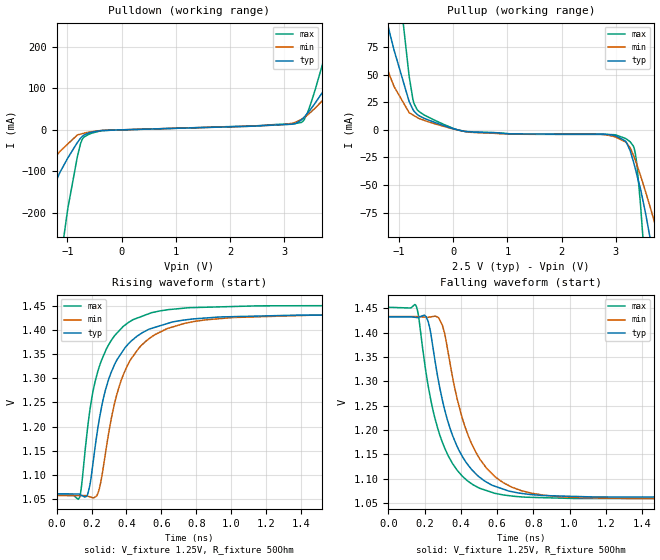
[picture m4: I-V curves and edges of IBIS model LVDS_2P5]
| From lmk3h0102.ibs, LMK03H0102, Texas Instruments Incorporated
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[Model]   LVDS_2P5
Model_type   Output
Polarity   Non-Inverting
Vmeas = 1.25
Vref = 1.25
Cref = 2pF
Rref = 50
|   typ   min   max
C_comp   2.5pF   2pF   3pF
[Voltage Range]   2.5   2.375   2.625
[Temperature Range]   45   125   -40
[Pullup Reference]   2.5   2.375   2.625
[Pulldown Reference]   -0   -0   -0
[Power Clamp Reference]   2.5   2.375   2.625
[GND Clamp Reference]   0   0   0
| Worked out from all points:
|   slope of the pulldown table from 0 to 0.375 V, typ, clamps not added: 278 ohm
|   slope of the pullup table from 0 to 0.375 V, typ, clamps not added: 121 ohm
|   falling waveform, V_fixture 1.25V, R_fixture 50Ohm: 20-80 % time 175ps typ, 189ps min, 158ps max; typ from 1.43 V to 1.06 V
|   rising waveform, V_fixture 1.25V, R_fixture 50Ohm: 20-80 % time 170ps typ, 188ps min, 145ps max; typ from 1.06 V to 1.43 V
[Pulldown]
|   Voltage   I(typ)   I(min)   I(max)
-3.3V     -897.3mA   -522.5mA   -2.711A
-2.181V   -448.8mA   -243.2mA   -1.452A
-1.617V   -265.6mA   -137.5mA   -832.1mA
-1.142V   -103.8mA   -52.61mA   -329.4mA
-993.3mV  -68.16mA   -34.35mA   -190.5mA
-815.1mV  -30.62mA   -12.44mA   -64.49mA
-706.2mV  -14.02mA   -8.857mA   -19.37mA
-389.4mV  -2.233mA   -2.057mA   -2.763mA
3.313V    22.93mA    24.44mA    17.28mA
3.937V    135.7mA    102mA      265.2mA
5.066V    387.9mA    287.8mA    848.7mA
6.6V      776.7mA    588.4mA    1.691A
[Pullup]
|   Voltage   I(typ)   I(min)   I(max)
-3.3V     558.8mA    397.8mA    1.302A
-1.607V   176.4mA    109.5mA    424.8mA
-1.092V   71.86mA    39mA       170.7mA
-666.6mV  13.84mA    11.09mA    18.07mA
66mV      6.39uA     -66.99uA   113.7uA
3.175V    -10.15mA   -10.88mA   -7.789mA
3.353V    -33.9mA    -26.75mA   -19.67mA
3.462V    -54.92mA   -42.4mA    -71.74mA
3.551V    -76.13mA   -56.4mA    -131.8mA
3.64V     -100mA     -71.05mA   -201.2mA
3.818V    -157.4mA   -102.3mA   -370.2mA
6.6V      -1.235A    -768.4mA   -3.496A
[Ramp]
R_load = 50
|   typ   min   max
dV/dt_r   0.223114/1.69348e-10   0.225528/1.86941e-10   0.236568/1.45415e-10
dV/dt_f   0.223109/1.74881e-10   0.225524/1.8824e-10   0.236568/1.57956e-10
[Falling Waveform]
V_fixture = 1.25V
V_fixture_min = 1.25V
V_fixture_max = 1.25V
R_fixture = 50Ohm
C_fixture = 0F
|   Time   V(typ)   V(min)   V(max)
0s        1.433V     1.433V     1.452V
154.3ps   1.431V     1.433V     1.455V
220.3ps   1.423V     1.432V     1.29V
277.7ps   1.299V     1.431V     1.197V
310ps     1.243V     1.4V       1.164V
339.2ps   1.205V     1.341V     1.141V
425.1ps   1.136V     1.205V     1.099V
588ps     1.084V     1.104V     1.07V
1.009ns   1.064V     1.062V     1.059V
5ns       1.061V     1.057V     1.058V
[Rising Waveform]
V_fixture = 1.25V
V_fixture_min = 1.25V
V_fixture_max = 1.25V
R_fixture = 50Ohm
C_fixture = 0F
|   Time   V(typ)   V(min)   V(max)
0s        1.061V     1.057V     1.058V
131.8ps   1.06V      1.057V     1.053V
179.1ps   1.061V     1.056V     1.202V
228.5ps   1.178V     1.056V     1.304V
254.8ps   1.235V     1.088V     1.335V
293.9ps   1.293V     1.177V     1.367V
366.3ps   1.349V     1.292V     1.401V
542.6ps   1.403V     1.385V     1.435V
1.009ns   1.427V     1.426V     1.448V
5ns       1.433V     1.433V     1.452V
